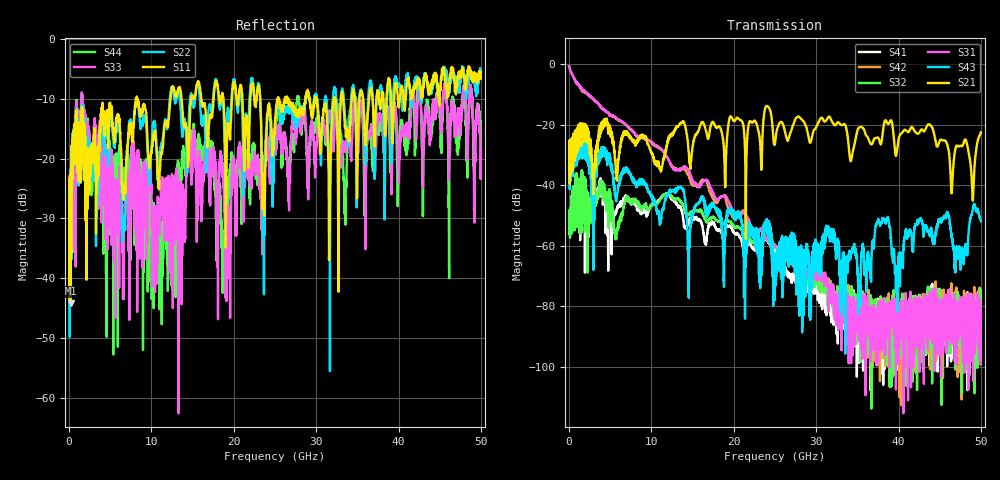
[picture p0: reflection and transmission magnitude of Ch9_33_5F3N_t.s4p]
!Agilent Technologies,N5247A,US51170199,A.09.90.13
!Agilent N5247A: A.09.90.13
!Date: Wednesday, December 16, 2015 11:01:44
!Correction: S11(Full 4 Port(1,2,3,4))
!S12(Full 4 Port(1,2,3,4))
!S13(Full 4 Port(1,2,3,4))
!S14(Full 4 Port(1,2,3,4))
!S21(Full 4 Port(1,2,3,4))
!S22(Full 4 Port(1,2,3,4))
!S23(Full 4 Port(1,2,3,4))
!S24(Full 4 Port(1,2,3,4))
!S31(Full 4 Port(1,2,3,4))
!S32(Full 4 Port(1,2,3,4))
!S33(Full 4 Port(1,2,3,4))
!S34(Full 4 Port(1,2,3,4))
!S41(Full 4 Port(1,2,3,4))
!S42(Full 4 Port(1,2,3,4))
!S43(Full 4 Port(1,2,3,4))
!S44(Full 4 Port(1,2,3,4))
!S4P File: Measurements: <S11,S12,S13,S14>,
!<S21,S22,S23,S24>,
!<S31,S32,S33,S34>,
!<S41,S42,S43,S44>:
# Hz S  dB  R 50
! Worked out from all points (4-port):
!   3201 points, 10 MHz to 50 GHz, reference 50 ohm
!   strongest paths, dB at 10 MHz, 12.51 GHz, 25 GHz, 37.5 GHz, 50 GHz:
!     S21: -34.4, -23.5, -26.4, -24.3, -22.6
!     S43: -34.7, -41.9, -63.6, -52.1, -51.9
!     S31: -0.7, -33.8, -60.1, -96.7, -82.1
!     S32: -55.4, -44.1, -60.3, -88.8, -78.5
!     S42: -0.8, -33.9, -60.5, -81.3, -77.4
!     S41: -55.9, -44.8, -61.8, -89.6, -83.1
!   lowest |S11| = -44.2 dB at 181.8 MHz (marker M1), VSWR 1.01, Z = 49.7 + j0.552 ohm
!   |S11| at or under -10 dB: start of sweep to 8.126 GHz; 8.253 GHz to 12.3 GHz (4.05 GHz wide, 39.4 % of centre); 23.21 GHz to 25.35 GHz (2.143 GHz wide, 8.82 % of centre)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
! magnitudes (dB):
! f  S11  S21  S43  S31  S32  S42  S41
! 10 MHz  -23.5  -34.4  -34.7  -0.7  -55.4  -0.8  -55.9
! 181.8 MHz  -44.2  -36.7  -38.7  -2.2  -48.0  -2.3  -48.6
! 12.12 GHz  -13.4  -24.7  -43.0  -31.8  -42.6  -31.9  -42.8
! 35.22 GHz  -10.7  -21.0  -73.5  -83.7  -78.4  -76.6  -89.4
! 37.47 GHz  -8.6  -24.3  -52.3  -91.0  -83.9  -80.9  -77.5
! 39.75 GHz  -7.5  -29.8  -72.6  -87.3  -86.3  -79.2  -85.3
! 50 GHz  -5.7  -22.6  -51.9  -82.1  -78.5  -77.4  -83.1
